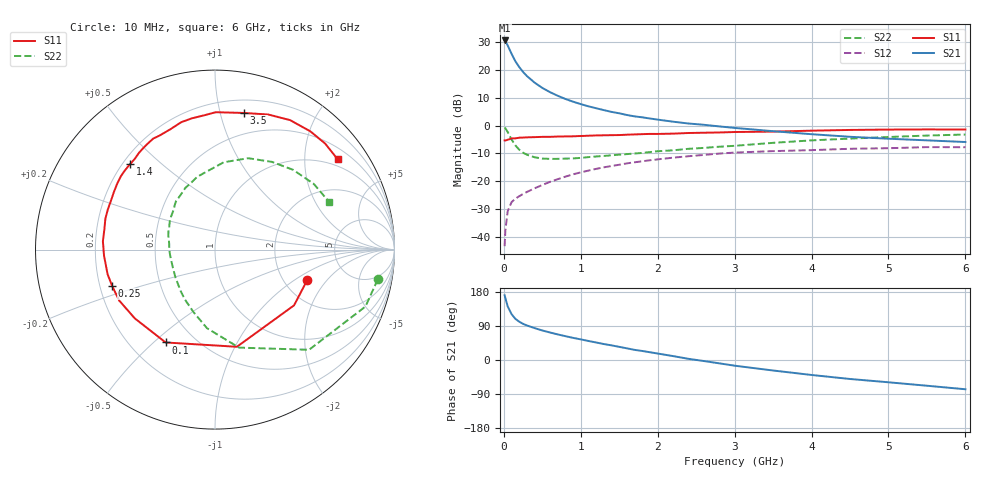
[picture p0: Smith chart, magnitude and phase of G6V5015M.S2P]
! SIEMENS Small Signal Semiconductors
! BFG193
! Si NPN RF Bipolar Junction Transistor in SOT223
! VCE = 0.5 V  IC = 15 mA
! Common Emitter S-Parameters:  August  1996
# GHz  S  MA  R  50
!  f  S11  S21  S12  S22
! GHz  MAG  ANG  MAG  ANG  MAG  ANG  MAG  ANG
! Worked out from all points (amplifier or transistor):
!   36 points, 10 MHz to 6 GHz, reference 50 ohm
!   highest |S21| = 30.6 dB at 10 MHz (marker M1)
!   |S21| within 3 dB of that: start of sweep to 70.37 MHz
!   unconditionally stable (mu >= 1): 600.2 MHz to 5.266 GHz; 5.595 GHz to end of sweep
!   at 250 MHz: K = 0.70, MSG = 21.9 dB, |S12| = -24.6 dB
!   at 1.4 GHz: K = 1.10, MAG = 7.8 dB, |S12| = -14.6 dB
!   at 6 GHz: K = 1.01, MAG = 0.3 dB, |S12| = -7.8 dB
!   S11 on the Smith chart (normalised r, x): 10 MHz: 2.67, -1.28; 100 MHz: 0.35, -0.55; 250 MHz: 0.25, -0.16; 1.4 GHz: 0.23, +0.40; 3.5 GHz: 0.31, +1.19; 6 GHz: 0.79, +2.85
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0.01  0.5414 -18.2  33.81 170.9  0.0068 84.6  0.9217 -10.4
0.02  0.5389 -35.2  32.68 163.3  0.0131 78.3  0.8965 -20.7
0.05  0.555 -77.3  27.55 141.4  0.0289 60.8  0.7657 -46.8
0.1  0.586 -118.0  19.51 121.1  0.042 49.5  0.5623 -76.2
0.15  0.5887 -139.4  14.29 108.6  0.0486 44.4  0.4403 -95.8
0.2  0.6046 -152.0  11.26 101.1  0.0537 44.0  0.3681 -109.0
0.25  0.6079 -160.6  9.172 95.4  0.059 44.5  0.3244 -121.2
0.3  0.6139 -167.1  7.753 91.1  0.0641 46.0  0.2992 -129.9
0.4  0.6191 -176.8  5.906 84.2  0.0745 47.5  0.2691 -145.2
0.5  0.6263 175.8  4.746 77.9  0.0855 48.0  0.2552 -156.7
0.6  0.6267 169.5  3.983 72.6  0.0973 48.8  0.2517 -165.4
0.7  0.6347 164.2  3.43 67.5  0.1087 48.5  0.2521 -173.1
0.8  0.6377 159.4  3.004 62.9  0.1207 47.4  0.255 179.9
1.1  0.6564 146.3  2.214 50.2  0.1551 43.8  0.2709 163.7
1.4  0.6717 134.6  1.759 38.6  0.1872 37.9  0.292 150.1
1.7  0.6931 125.1  1.462 26.7  0.2187 32.0  0.3144 138.5
2.2  0.7153 110.3  1.173 10.3  0.2647 20.2  0.3591 122.5
2.8  0.7508 94.5  0.965 -8.8  0.3137 6.3  0.4167 104.0
3.5  0.7783 78.0  0.792 -27.7  0.3473 -11.2  0.4889 84.3
4.5  0.8339 59.9  0.628 -50.1  0.3826 -29.8  0.5827 57.0
5.5  0.8519 43.9  0.542 -67.9  0.4096 -51.3  0.661 33.6
6  0.8486 36.3  0.506 -77.2  0.4078 -63.5  0.6898 22.5
